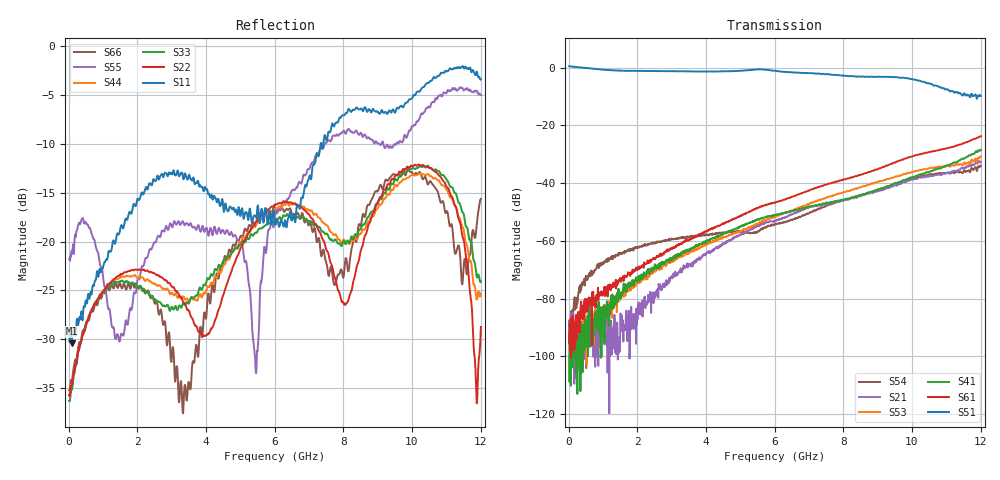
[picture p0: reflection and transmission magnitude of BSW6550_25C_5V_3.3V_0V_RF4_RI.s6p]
! Agilent Technologies	N5230C	MY49001333	A.09.33.09
!	Test time	=	2026-05-06 10:00
!	Product	=	BSW6550
!	Temp	=	25C
!	VDD	=	5
!	Control_High	=	3.3
!	Control_Low	=	0
!	Logic	=	RF4
!	Port1	=	RFC
!	Port2	=	RF1
!	Port3	=	RF2
!	Port4	=	RF3
!	Port5	=	RF4
!	Port6	=	RF5
!	V1	=	3.3 / 0
!	V2	=	3.3 / 0
!	V3	=	3.3 / 0
!S6P File: Measurements: <S11,S12,S13,S14,S15,S16>,
!<S21,S22,S23,S24,S25,S26>,
!<S31,S32,S33,S34,S35,S36>,
!<S41,S42,S43,S44,S45,S46>,
!<S51,S52,S53,S54,S55,S56>,
!<S61,S62,S63,S64,S65,S66>;
# HZ S RI R 50
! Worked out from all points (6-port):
!   1201 points, 10 MHz to 12.01 GHz, reference 50 ohm
!   strongest paths, dB at 10 MHz, 3.01 GHz, 6.01 GHz, 9.01 GHz, 12.01 GHz:
!     S51: 0.5, -1.3, -1.1, -3.2, -9.8
!     S61: -95.3, -62.9, -46.8, -35.2, -23.8
!     S41: -108.6, -66.0, -51.1, -42.2, -28.5
!     S53: -93.4, -66.7, -51.5, -39.6, -31.0
!     S21: -91.8, -72.7, -53.1, -42.8, -32.6
!     S54: -89.5, -59.5, -54.1, -42.3, -34.1
!   lowest |S11| = -30.4 dB at 90 MHz (marker M1), VSWR 1.06, Z = 53 - j0.607 ohm
!   |S11| at or under -10 dB: start of sweep to 7.343 GHz; 7.363 GHz to 7.419 GHz (56.63 MHz wide, 0.766 % of centre)
